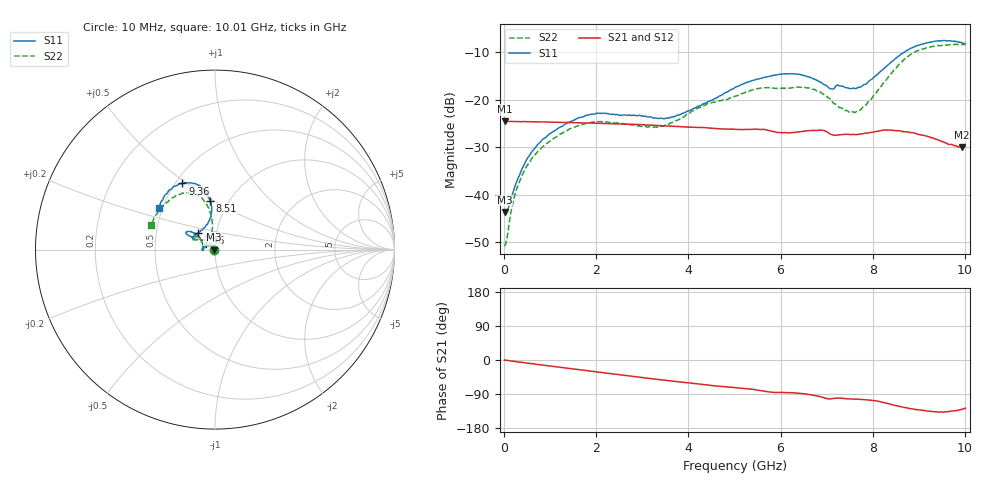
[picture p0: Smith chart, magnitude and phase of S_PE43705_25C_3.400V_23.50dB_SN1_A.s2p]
! Device ID: PE43705
! Serial: 1
! Insertion: A
! Impedance: 50 ohm
! Temp: 25C
! VDD: 3.400V
! Attenuation Step: 23.50dB
#  Hz  S  RI  R  50
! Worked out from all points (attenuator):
!   401 points, 10 MHz to 10.01 GHz, reference 50 ohm
!   highest |S21| = -24.54 dB at 10 MHz (marker M1); lowest = -29.9 dB at 9.935 GHz (marker M2)
!   lowest |S11| = -43.6 dB at 10 MHz (marker M3), VSWR 1.01, Z = 49.3 + j0.0433 ohm
!   |S11| at or under -10 dB: start of sweep to 8.683 GHz
!   |S22| runs from -50.8 to -8.3 dB; largest |S21 - S12| = 0.00081
!   S11 on the Smith chart (normalised r, x): 10 MHz: 0.99, +0.00; 7.46 GHz: 0.81, +0.16; 8.51 GHz: 0.82, +0.48; 9.36 GHz: 0.54, +0.48; 10.01 GHz: 0.48, +0.26
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1e7  -0.00658 0.000439  0.0593 -0.000227  0.0593 -0.000222  -0.00285 0.000487
8.5e7  -0.00624 0.00347  0.0591 -0.0015  0.0591 -0.00148  -0.0023 0.00337
2.6e8  -0.00774 0.0109  0.0588 -0.00444  0.0587 -0.0044  -0.0036 0.0105
5.35e8  -0.0147 0.0207  0.058 -0.0089  0.058 -0.00888  -0.00961 0.0192
1.01e9  -0.0356 0.0265  0.0558 -0.0162  0.0559 -0.0161  -0.0278 0.0245
1.685e9  -0.0636 0.0161  0.0511 -0.0254  0.0512 -0.0253  -0.0523 0.0168
2.16e9  -0.072 0.00248  0.0468 -0.0313  0.0469 -0.0312  -0.0578 0.00709
3.36e9  -0.0634 0.00268  0.0332 -0.0419  0.0331 -0.0418  -0.0501 0.0129
3.86e9  -0.0668 0.0253  0.0271 -0.0444  0.0271 -0.0443  -0.0586 0.0278
5.01e9  -0.1039 0.0854  0.0143 -0.0468  0.0144 -0.0467  -0.0888 0.0634
5.535e9  -0.1335 0.0981  0.00837 -0.048  0.00837 -0.0481  -0.1082 0.0745
6.01e9  -0.1565 0.099  0.0036 -0.045  0.00374 -0.0448  -0.1105 0.0714
6.685e9  -0.148 0.0787  -0.00211 -0.0475  -0.00233 -0.0474  -0.1145 0.0589
7.085e9  -0.1152 0.0611  -0.00936 -0.0423  -0.0094 -0.0423  -0.0844 0.0557
7.46e9  -0.0943 0.0941  -0.00936 -0.0422  -0.00916 -0.0422  -0.0499 0.0574
7.785e9  -0.0515 0.1319  -0.0108 -0.0425  -0.0106 -0.0424  -0.0275 0.0791
8.36e9  -0.0185 0.2387  -0.0208 -0.0432  -0.0207 -0.0433  -0.0197 0.1785
8.51e9  -0.0274 0.2733  -0.024 -0.0409  -0.024 -0.0407  -0.0305 0.2147
8.91e9  -0.0814 0.3532  -0.0288 -0.034  -0.0285 -0.0341  -0.0966 0.302
9.36e9  -0.1817 0.3687  -0.0279 -0.0263  -0.0284 -0.0265  -0.1984 0.3074
9.935e9  -0.3054 0.2544  -0.0204 -0.0244  -0.0205 -0.0246  -0.3433 0.1653
1.001e10  -0.3144 0.2297  -0.0193 -0.0259  -0.0201 -0.0258  -0.3582 0.1361
